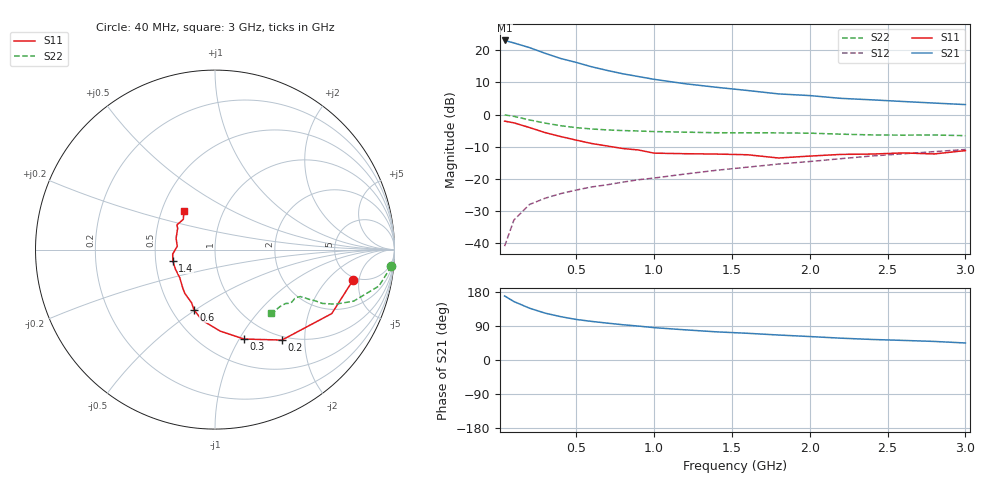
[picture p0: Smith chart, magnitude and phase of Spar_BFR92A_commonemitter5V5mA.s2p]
! Filename:  BFR92AB.S2P  Version:  2.0
! NXP part #: BFR92A  Date: May 1990
! Bias condition: Vce=5V, Ic=5mA
#  MHz  S  MA  R  50
! Freq  S11  S21  S12  S22  !GUM [dB]
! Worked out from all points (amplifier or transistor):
!   21 points, 40 MHz to 3 GHz, reference 50 ohm
!   highest |S21| = 23.0 dB at 40 MHz (marker M1)
!   |S21| within 3 dB of that: start of sweep to 244 MHz
!   unconditionally stable (mu >= 1): 1.159 GHz to 2.835 GHz
!   at 300 MHz: K = 0.51, MSG = 22.5 dB, |S12| = -26.0 dB
!   at 1 GHz: K = 0.98, MSG = 15.3 dB, |S12| = -19.7 dB
!   at 3 GHz: K = 0.98, MSG = 7.0 dB, |S12| = -10.9 dB
!   S11 on the Smith chart (normalised r, x): 40 MHz: 4.71, -4.16; 200 MHz: 0.94, -1.56; 300 MHz: 0.76, -1.05; 600 MHz: 0.64, -0.49; 1.4 GHz: 0.62, -0.08; 3 GHz: 0.65, +0.30
40  0.789 -12.2  14.15 169.0  0.009 85.7  0.987 -5.4
100  0.742 -28.7  12.94 154.2  0.023 74.9  0.936 -12.5
200  0.627 -53.5  10.95 136.7  0.04 66.9  0.824 -20.4
300  0.524 -72.0  8.943 123.7  0.05 62.6  0.736 -24.4
400  0.455 -86.4  7.427 114.4  0.059 60.9  0.67 -26.6
500  0.4 -100.5  6.449 107.0  0.067 60.8  0.625 -27.1
600  0.354 -109.4  5.509 101.8  0.075 62.4  0.596 -27.8
700  0.324 -113.7  4.835 97.3  0.081 63.9  0.576 -28.1
800  0.296 -124.7  4.293 93.0  0.089 64.8  0.563 -28.3
900  0.281 -129.5  3.89 89.5  0.097 66.0  0.555 -28.6
1000  0.251 -141.5  3.524 85.4  0.103 67.3  0.543 -28.8
1200  0.246 -153.8  3.007 79.6  0.119 68.9  0.532 -29.8
1400  0.243 -165.3  2.651 74.3  0.136 69.1  0.521 -31.5
1600  0.237 -174.0  2.363 70.5  0.152 71.0  0.52 -32.6
1800  0.211 174.9  2.091 65.9  0.17 71.2  0.518 -34.3
2000  0.226 163.6  1.969 61.9  0.186 71.6  0.513 -35.7
2200  0.24 149.9  1.783 57.6  0.206 72.3  0.495 -37.3
2400  0.243 149.5  1.69 54.2  0.227 71.5  0.482 -40.9
2600  0.253 146.9  1.593 51.7  0.245 71.1  0.478 -44.4
2800  0.244 136.4  1.506 49.0  0.265 71.1  0.481 -46.9
3000  0.275 129.0  1.427 44.9  0.286 70.2  0.469 -48.4
